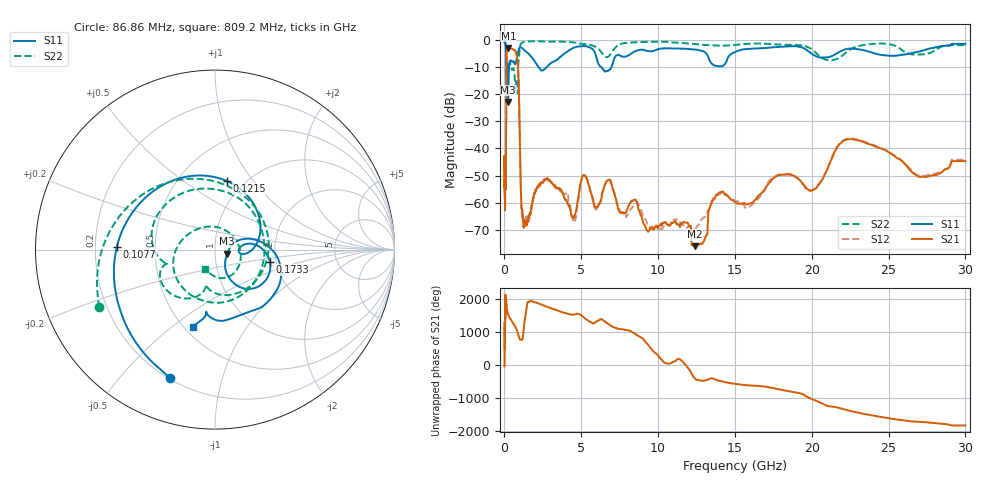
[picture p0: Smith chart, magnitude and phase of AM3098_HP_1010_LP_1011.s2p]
! Date/Time: Thu, Feb 28, 2019 8:42 AM
! Network Analyzer: Agilent Technologies E8364B Rev: A.07.50.67
! Sweep from 0.010 to 30.000 GHz, 1601 Points, Sweep Type: LOG
! Power Supply: 5.022 V, 0.002 A
# Hz S DB R 50
!freq MagS11 AngS11 MagS21 AngS21 MagS12 AngS12 MagS22 AngS22
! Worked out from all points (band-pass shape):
!   1601 points, 10 MHz to 30 GHz, reference 50 ohm
!   highest |S21| = -3.11 dB at 252.2 MHz (marker M1); lowest = -76.0 dB at 12.37 GHz (marker M2)
!   |S21| within 3 dB of the highest: 133.9 MHz to 806.4 MHz (672.5 MHz wide, 143 % of centre)
!   lowest |S11| = -22.9 dB at 241.1 MHz (marker M3), VSWR 1.15, Z = 57.2 - j2.5 ohm
!   |S11| at or under -10 dB: 192.2 MHz to 303.4 MHz (111.2 MHz wide, 44.9 % of centre); 2.196 GHz to 2.779 GHz (582.2 MHz wide, 23.4 % of centre); 6.257 GHz to 6.975 GHz (718.6 MHz wide, 10.9 % of centre)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
!   |S22| runs from -19.9 to -0.6 dB; largest |S21 - S12| = 0.013
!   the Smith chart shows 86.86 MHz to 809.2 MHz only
!   S11 on the Smith chart (normalised r, x): 86.86 MHz: 0.21, -0.69; 107.7 MHz: 0.29, +0.01; 121.5 MHz: 0.83, +0.75; 173.3 MHz: 1.85, -0.28; 809.2 MHz: 0.55, -0.59
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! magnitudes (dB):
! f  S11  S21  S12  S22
! 10 MHz  -0.3  -42.9  -42.9  -0.6
! 38.04 MHz  -0.5  -60.3  -58.8  -0.9
! 86.86 MHz  -2.4  -54.4  -53.0  -2.9
! 107.7 MHz  -5.2  -31.5  -31.2  -6.6
! 121.5 MHz  -8.2  -12.8  -12.8  -10.6
! 144.7 MHz  -17.6  -4.7  -4.7  -13.8
! 173.3 MHz  -10.1  -3.9  -3.9  -9.5
! 241.1 MHz  -22.9  -3.1  -3.1  -11.2
! 252.2 MHz  -20.3  -3.1  -3.1  -11.0
! 550.5 MHz  -8.0  -3.7  -3.6  -10.6
! 809.2 MHz  -7.0  -6.2  -6.2  -18.4
! 921.7 MHz  -3.9  -15.0  -15.0  -7.6
! 1.143 GHz  -3.2  -62.6  -64.9  -1.2
! 2.084 GHz  -8.9  -55.0  -55.2  -0.6
! 4.503 GHz  -3.0  -65.7  -67.1  -1.0
! 5.206 GHz  -2.4  -50.0  -49.6  -1.7
! 7.926 GHz  -6.2  -63.4  -65.3  -1.2
! 12.37 GHz  -3.7  -76.0  -69.5  -1.6
! 13.95 GHz  -9.9  -56.4  -57.0  -2.3
! 20.1 GHz  -5.6  -55.2  -55.3  -4.1
! 22.44 GHz  -3.4  -36.6  -36.4  -3.9
! 30 GHz  -1.6  -44.7  -44.2  -2.1
